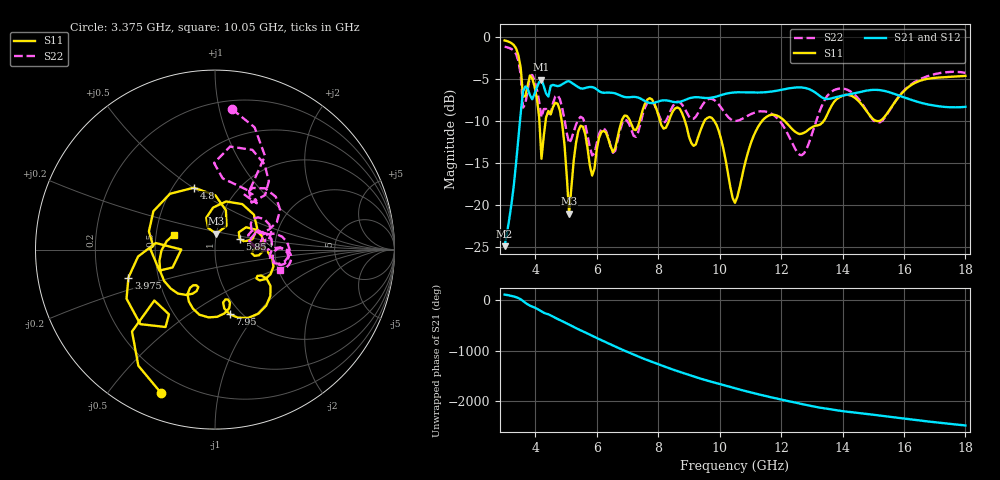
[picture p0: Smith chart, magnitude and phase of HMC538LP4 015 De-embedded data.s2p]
! Chelmsford, MA 01824
! http://www.hittite.com
! Tel: 978-250-3343
! Fax: 978-250-3373
! Device  :  HMC538LP4
! Description:  600 Analog Phase Shifter
! Frequency  :  6.0 GHz - 15.0 GHz
! Package  :  LP4  - 4x4 mm Quad Flatpack No-Lead (QFN) Plastic Package: 24 pin
! Ports  :  2 RF, 1 DC
!  Pin  3  = Rfin  = Port 1
!  Pin  16  = Rfout = Port 2
!  pin  21  = vCTL
! Voltages:  VCTL  = 0 to 5.0 Volts
! Currents :  Vb(V)  Vd(V)  Ib(mA)  Id(mA)
!  0.00  1.50  0.000000	0.489095
! Data:  The device was measured on evaluation board 111296-1.
!  Data was collected using a calibrated network analyzer.
!  The evaluation circuit board was modeled and simulated.This was use
!  to removed the evaluation board circuit from the measured data.
!  The reference plane is the center of the package pin.
! Misc:  Lot #
!Date Measured:  03 - 11 -2009
! Date:  03 - 17 -2009
! Note:
!  Hittite Microwave supplies this data as a sample of measured data at the
!  package pin for this package product.  Your particular data for this product
!  may vary.
!  Data was taken at 25 degrees C.
!  Hittite Microwave reserves the right to change this data at anytime.
# MHz S MA R 50
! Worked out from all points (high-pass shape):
!   201 points, 3 GHz to 18 GHz, reference 50 ohm
!   highest |S21| = -5.10 dB at 4.2 GHz (marker M1); lowest = -24.9 dB at 3 GHz (marker M2)
!   |S21| within 3 dB of the highest: 3.553 GHz to 16.84 GHz (13.29 GHz wide, 130 % of centre)
!   lowest |S11| = -21.1 dB at 5.1 GHz (marker M3), VSWR 1.19, Z = 49.9 + j8.88 ohm
!   |S11| at or under -10 dB: 4.857 GHz to 6.814 GHz (1.957 GHz wide, 33.5 % of centre); 9.821 GHz to 11.39 GHz (1.568 GHz wide, 14.8 % of centre); 12.11 GHz to 13.39 GHz (1.285 GHz wide, 10.1 % of centre)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
!   |S22| runs from -14.1 to -1.2 dB; largest |S21 - S12| = 0.0013
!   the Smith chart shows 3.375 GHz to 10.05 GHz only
!   S11 on the Smith chart (normalised r, x): 3.375 GHz: 0.12, -0.68; 3.975 GHz: 0.33, -0.14; 4.8 GHz: 0.63, +0.50; 5.85 GHz: 1.31, +0.16; 7.95 GHz: 0.89, -0.74; 10.05 GHz: 0.62, +0.11
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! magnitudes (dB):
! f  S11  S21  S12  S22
! 3 GHz  -0.4  -24.9  -24.9  -1.2
! 3.375 GHz  -1.4  -15.0  -15.0  -2.1
! 3.6 GHz  -7.1  -6.5  -6.5  -8.4
! 3.975 GHz  -5.9  -6.8  -6.8  -5.2
! 4.2 GHz  -14.5  -5.1  -5.1  -9.6
! 4.425 GHz  -8.8  -7.1  -7.1  -9.2
! 4.8 GHz  -8.8  -5.8  -5.8  -7.4
! 5.1 GHz  -21.1  -5.3  -5.3  -12.7
! 5.55 GHz  -10.7  -6.2  -6.2  -9.7
! 5.85 GHz  -16.5  -6.0  -6.0  -14.1
! 6.15 GHz  -11.3  -6.6  -6.6  -11.0
! 6.525 GHz  -13.7  -6.7  -6.7  -13.8
! 7.95 GHz  -8.7  -7.8  -7.8  -8.7
! 8.025 GHz  -9.6  -7.7  -7.7  -9.4
! 10.05 GHz  -12.2  -6.9  -7.0  -8.4
! 10.5 GHz  -19.8  -6.6  -6.6  -10.0
! 11.47 GHz  -9.7  -6.6  -6.6  -8.9
! 12.6 GHz  -11.6  -6.0  -6.0  -14.0
! 13.05 GHz  -10.7  -6.5  -6.5  -11.1
! 13.88 GHz  -7.3  -7.1  -7.1  -6.2
! 15.53 GHz  -8.7  -6.6  -6.6  -8.8
! 18 GHz  -4.7  -8.3  -8.3  -4.3
